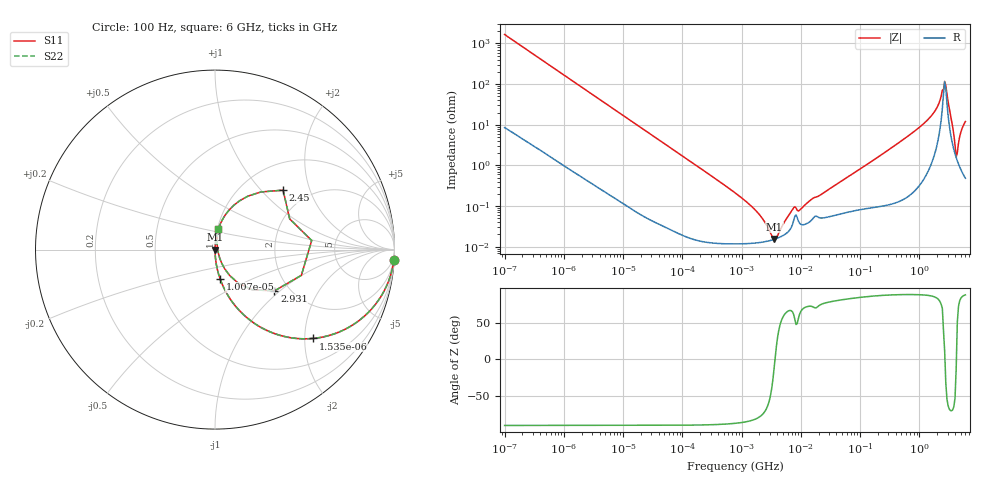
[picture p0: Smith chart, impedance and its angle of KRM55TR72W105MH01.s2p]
!Murata Part Number: KRM55TR72W105MH01
!These Parameters are Measured in Series Mode Connection
!Data Generated on Jan 08, 2026
!  o--ll--o
!Port1  Port2
!  o------o
!Operation Temp=25[degC], DC Bias Voltage=0[V]
!Freq. Start=100[Hz] Stop=6[GHz] 401[Steps]
# Hz S RI R 50
!Freq.(Hz) S11(Real) S11(Imag) S21(Real) S21(Imag) S12(Real) S12(Imag) S22(Real) S22(Imag)
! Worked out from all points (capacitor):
!   401 points, 100 Hz to 6 GHz, reference 50 ohm
!   read as one part in series: C = 953 nF near 109 Hz
!   lowest |Z| = 15.4 mohm at 3.55 MHz (marker M1)
!   series resonance near 3.667 MHz, so ESL is about 2 nH
!   S11 on the Smith chart (normalised r, x): 100 Hz: 1, -33; 1.535 kHz: 1.01, -2.19; 10.07 kHz: 1.00, -0.34; 2.45 GHz: 1.51, +1.34; 2.931 GHz: 1.67, -0.92; 6 GHz: 1.01, +0.24
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100  0.9961 -0.0597  0.00389 0.0597  0.00389 0.0597  0.9961 -0.0597
524  0.9097 -0.2837  0.0903 0.2837  0.0903 0.2837  0.9097 -0.2837
1535  0.5459 -0.4949  0.4541 0.4949  0.4541 0.4949  0.5459 -0.4949
2008  0.4139 -0.4895  0.5861 0.4895  0.5861 0.4895  0.4139 -0.4895
4299  0.1356 -0.3391  0.8644 0.3391  0.8644 0.3391  0.1356 -0.3391
10066  0.0287 -0.1636  0.9713 0.1636  0.9713 0.1636  0.0287 -0.1636
40335  0.00214 -0.0422  0.9979 0.0422  0.9979 0.0422  0.00214 -0.0422
774597  0.000121 -0.00212  0.9999 0.00212  0.9999 0.00212  0.000121 -0.00212
1896632  0.000125 -0.000661  0.9999 0.000661  0.9999 0.000661  0.000125 -0.000661
3549919  0.000151 -3.01e-05  0.9998 3.01e-05  0.9998 3.01e-05  0.000151 -3.01e-05
7266822  0.000358 0.000748  0.9996 -0.000748  0.9996 -0.000748  0.000358 0.000748
9506416  0.00038 0.000687  0.9996 -0.000687  0.9996 -0.000687  0.00038 0.000687
1.555665e7  0.00047 0.00143  0.9995 -0.00143  0.9995 -0.00143  0.00047 0.00143
3.124326e8  0.0017 0.0248  0.9983 -0.0248  0.9983 -0.0248  0.0017 0.0248
1.712697e9  0.047 0.1766  0.953 -0.1766  0.953 -0.1766  0.047 0.1766
2.450438e9  0.3793 0.3311  0.6207 -0.3311  0.6207 -0.3311  0.3793 0.3311
2.931063e9  0.3314 -0.23  0.6686 0.23  0.6686 0.23  0.3314 -0.23
3.352442e9  0.0818 -0.1444  0.9182 0.1444  0.9182 0.1444  0.0818 -0.1444
4.193612e9  0.0154 -0.00335  0.9846 0.00335  0.9846 0.00335  0.0154 -0.00335
4.586474e9  0.0118 0.0325  0.9882 -0.0325  0.9882 -0.0325  0.0118 0.0325
5.245841e9  0.013 0.0775  0.987 -0.0775  0.987 -0.0775  0.013 0.0775
6e9  0.0188 0.1171  0.9812 -0.1171  0.9812 -0.1171  0.0188 0.1171
